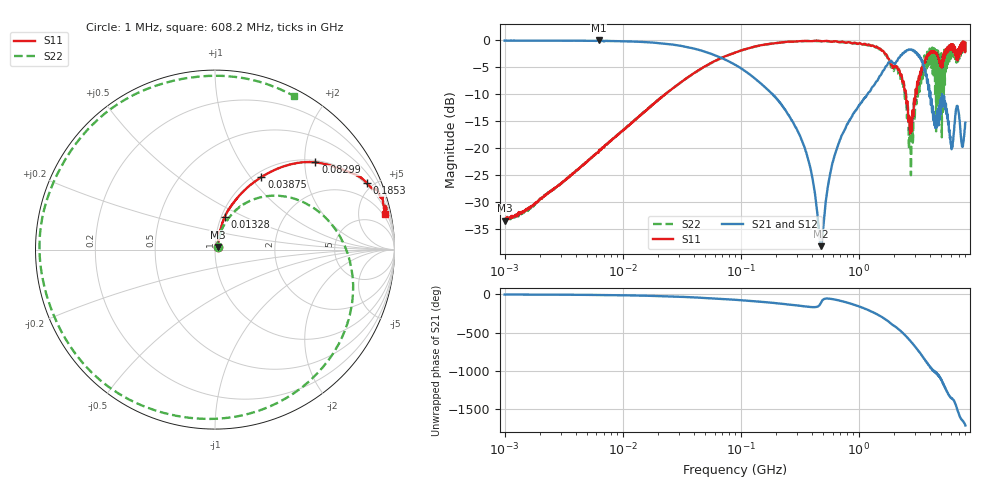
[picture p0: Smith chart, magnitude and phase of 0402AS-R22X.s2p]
!s-Parameter Generated by FASTRON Sdn. Bhd.
!FASTRON P/N : 0402AS-R22X
!Keysight Technologies: E5071C_MY46733604_B.14.02
!Date: Mon Dec 01 10:50:21 2025
!Version  :Rev00  Mon Dec 01 10:50:21 2025
!Data & Calibration Information:
!Freq  S11:SOLT2(ON)  S21:SOLT2(ON)  S12:SOLT2(ON)  S22:SOLT2(ON)
!PortZ  Port1:50+j0  Port2:50+j0
!When reading reference impedance value at option line is always used.
! Remarks : This data is being provided solely for informational purposes.
# Hz S dB R 50
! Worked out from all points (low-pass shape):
!   1601 points, 1 MHz to 8 GHz, reference 50 ohm
!   highest |S21| = -0.11 dB at 6.268 MHz (marker M1); lowest = -38.1 dB at 478.4 MHz (marker M2)
!   |S21| within 3 dB of the highest: start of sweep to 65 MHz; 2.234 GHz to 3.222 GHz (987.7 MHz wide, 36.2 % of centre)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
!   lowest |S11| = -33.4 dB at 1.013 MHz (marker M3), VSWR 1.04, Z = 51.5 + j1.57 ohm
!   |S11| at or under -10 dB: start of sweep to 23.05 MHz; 2.505 GHz to 3.02 GHz (515 MHz wide, 18.6 % of centre); 3.08186 GHz to 3.08186 GHz (0 Hz wide, 0 % of centre)
!   |S22| runs from -33.4 to -0.2 dB; largest |S21 - S12| = 0.014
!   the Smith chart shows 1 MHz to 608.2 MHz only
!   S11 on the Smith chart (normalised r, x): 1 MHz: 1.03, +0.03; 13.28 MHz: 1.04, +0.39; 38.75 MHz: 1.08, +1.13; 82.99 MHz: 1.05, +2.26; 185.3 MHz: 0.91, +4.61; 608.2 MHz: 1.56, +9.34
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1000000  -33.20 44.9  -0.14 -1.1  -0.13 -1.1  -33.20 43.0
1013202  -33.40 45.3  -0.14 -1.1  -0.13 -1.1  -33.40 45.0
4479405  -23.30 73.1  -0.17 -4.8  -0.16 -4.8  -23.30 71.2
6268472  -20.80 73.8  -0.11 -6.5  -0.11 -6.9  -20.70 72.5
1.328499e7  -14.40 73.4  -0.34 -14.1  -0.35 -14.1  -14.40 66.6
2.00676e7  -11.10 68.6  -0.59 -20.8  -0.59 -20.7  -11.10 59.4
3.87485e7  -6.38 57.4  -1.53 -37.3  -1.53 -37.2  -6.41 38.5
8.299405e7  -2.60 41.0  -4.20 -66.2  -4.19 -66.2  -2.62 -1.9
8.994653e7  -2.33 38.9  -4.62 -69.9  -4.61 -70.0  -2.33 -7.3
1.852822e8  -0.69 23.6  -10.00 -109.0  -10.00 -109.0  -0.69 -69.2
4.006501e8  -0.24 13.7  -25.00 -165.0  -25.00 -165.0  -0.19 170.0
4.783555e8  -0.26 14.1  -38.10 -108.0  -38.00 -108.0  -0.22 130.0
6.082397e8  -0.30 11.9  -22.20 -62.7  -22.20 -62.8  -0.34 62.6
8.899672e8  -0.63 11.5  -13.80 -129.0  -13.80 -129.0  -0.62 -79.9
1.075264e9  -0.86 14.2  -11.30 -173.0  -11.30 -173.0  -0.80 -173.0
1.249007e9  -1.03 18.0  -9.46 145.0  -9.47 145.0  -1.01 99.9
1.457824e9  -1.56 20.2  -7.29 94.6  -7.29 94.5  -1.46 -2.0
1.7949e9  -3.49 21.8  -4.14 2.9  -4.16 2.8  -3.84 -178.0
2.486897e9  -9.29 32.5  -2.15 -179.0  -2.14 -179.0  -10.10 -170.0
3.102129e9  -9.18 141.0  -2.57 10.1  -2.56 9.8  -9.20 -1.1
3.730463e9  -3.52 142.0  -6.29 -156.0  -6.29 -157.0  -3.75 53.6
8e9  -0.55 -94.0  -15.30 87.1  -15.30 86.8  -2.25 149.0
